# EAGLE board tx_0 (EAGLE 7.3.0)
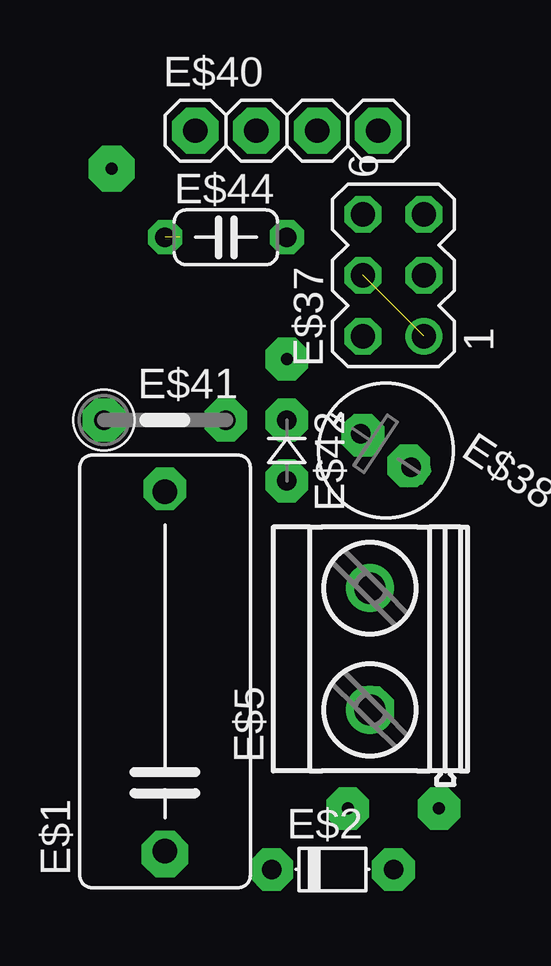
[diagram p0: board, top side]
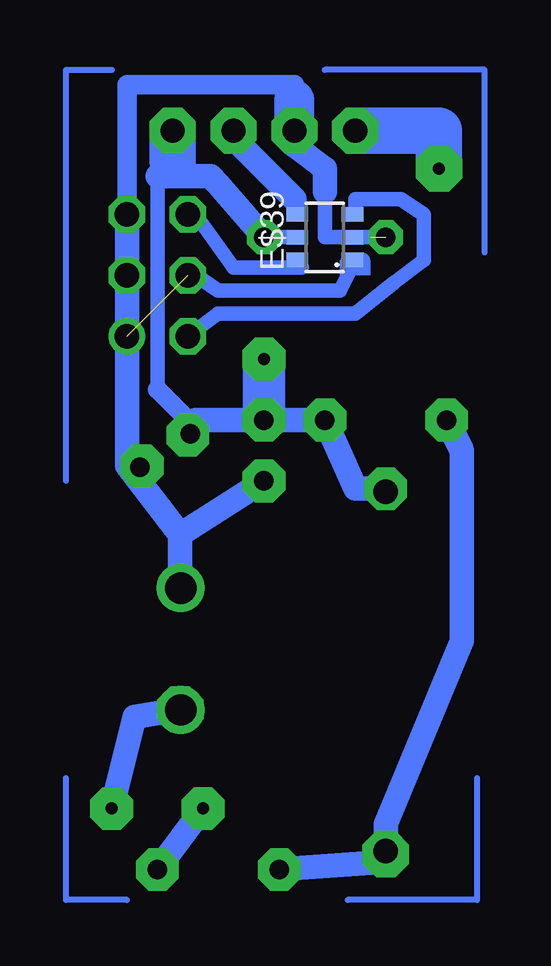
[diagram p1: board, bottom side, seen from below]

No outline drawn. Coordinates in mm, seen from the top.
Copper layers (1*16): Top 0.035mm / dielectric 1.5mm / Bottom 0.035mm
Design rules "default": minimum track width 10mil, minimum drill 24mil, track to track 8mil, track to pad 8mil, pad to pad 8mil, via to via 8mil, smd to smd 8mil, copper to edge 40mil, drill to drill 8mil, minimum pad ring 10mil, minimum via ring 8mil, stop-mask expansion 4mil, vias tented up to drill 0mil, thermal gap 10mil

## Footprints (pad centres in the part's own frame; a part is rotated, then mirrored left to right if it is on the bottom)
C150-072X183 = drill 1.016 octagon: 1 -7.493,0; 2 7.493,0
D-5 = drill 0.813 octagon: A 2.54,0; C -2.54,0
MKDSN1,5/2-5,08 = drill 1.3 pad 2: 1 -2.561,0.025; 2 2.519,0.025
MA03-2 = drill 1.016: 1 -2.54,-1.27 | drill 1.016 octagon: 2 -2.54,1.27; 3 0,-1.27; 4 0,1.27; 5 2.54,-1.27; 6 2.54,1.27
E2,5-6E = drill 0.813 pad 1.575: + -1.27,0 | drill 0.813 pad 1.575 octagon: - 1.27,0
SOT23-6 = smd 0.6 x 0.9: 1 -0.95,-1.15; 2 0,-1.15; 3 0.95,-1.15; 4 0.95,1.15; 5 0,1.15; 6 -0.95,1.15
1X04 = drill 1.016 octagon: 1 -3.81,0; 2 -1.27,0; 3 1.27,0; 4 3.81,0
0207/5V = drill 0.813 octagon: 1 -2.54,0; 2 2.54,0
D-2.5 = drill 0.813 octagon: A 1.27,0; C -1.27,0
C050-024X044 = drill 0.813 octagon: 1 -2.54,0; 2 2.54,0

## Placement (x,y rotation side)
E$1  [C150-072X183]  -13.02,27.94 90 top
E$2  [D-5]  -6.03,19.68 0 top
E$5  [MKDSN1,5/2-5,08]  -4.45,28.89 90 top
E$37  [MA03-2]  -3.49,44.45 90 top
E$38  [E2,5-6E]  -3.81,37.15 326.3 top
E$39  [SOT23-6]  -10.48,46.04 90 bottom
E$40  [1X04]  -7.94,50.48 0 top
E$41  [0207/5V]  -13.02,38.42 0 top
E$42  [D-2.5]  -7.94,37.15 270 top
E$44  [C050-024X044]  -10.48,46.04 0 top

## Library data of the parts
E$1 E$38 E$41 E$44 = rcl
E$2 E$42 = diode
E$5 = con-phoenix-508
E$37 = con-lstb
E$39 = microchip
E$40 = pinhead_hex

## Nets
S$128: E$37.6
S$129: E$37.4
S$130: E$37.2
S$139: E$38.+
S$158: E$42.A
S$162: E$37.5 E$38.-

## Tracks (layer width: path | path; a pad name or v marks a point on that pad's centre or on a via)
S$125
  Bottom 1.016: -15.56,38.42 -16.19,37.15 -16.19,29.21 -13.02,21.59 -13.02,20 -8.57,19.68
S$126  (via drill 0.5 pad 1.93)
  Bottom 1.93: v-15.24,48.9 -15.24,50.48 -11.75,50.48
S$127
  Bottom 0.61: -9.21,47.62 -9.21,46.99 | -6.67,50.16 -6.67,50.48
  Bottom 1.016: -9.21,47.62 -6.67,50.16
S$128
  Bottom 0.61: -9.53,44.77 -6.67,44.77 -5.08,46.99 E$37.6
S$129
  Bottom 0.61: -11.75,45.09 -11.11,43.81 -6.03,43.81 -5.08,44.45 E$37.4
S$130
  Bottom 0.61: -11.75,46.99 -11.75,47.62 -13.65,47.62 -14.61,46.99 -14.61,45.09 -13.34,44.13 -11.75,42.86 -6.03,42.86 E$37.2
S$131  (via drill 0.5 pad 1.93)
  other vias: -13.02,20.32
S$132  (via drill 0.5 pad 1.78, 0.5 pad 1.93)
  Bottom 1.016: v-4.45,26.35 -2.54,26.04 v-1.59,22.23
S$133  (via drill 0.5 pad 1.42)
  other vias: -4.76,41.91
S$135  (via drill 0.5 pad 1.78)
  other vias: -13.02,35.56
S$136  (via drill 0.5 pad 1.78)
  other vias: -10.48,38.42
S$137  (via drill 0.5 pad 1.78)
  other vias: -4.76,37.78
S$138  (via drill 0.5 pad 1.93)
  other vias: -6.67,50.48
S$139  (via drill 0.5 pad 1.93)
  Bottom 0.61: -3.49,39.69 -3.49,48.58 | -7.94,46.04 -9.21,46.04
  Bottom 0.813: -3.49,48.58 -4.13,48.58 -4.13,49.21 | -5.08,38.1 -3.49,39.69
  Bottom 1.016: -7.94,46.04 -6.03,48.26 -5.71,48.58 -3.49,48.58 | E$38.+ -5.08,38.1 -5.08,38.42 -10.48,38.42 -11.75,35.56 -13.02,35.56
  Bottom 1.778: -4.13,49.53 -4.13,49.21
  Bottom 1.93: -4.13,49.53 v-4.13,50.48 -4.13,49.21
S$140  (via drill 0.5 pad 1.93)
  other vias: -9.21,50.48
S$141  (via drill 0.5 pad 1.93)
  other vias: -11.75,50.48
S$142  (via drill 0.5 pad 1.42)
  other vias: -2.22,46.99
S$143  (via drill 0.5 pad 1.42)
  other vias: -4.76,46.99
S$144  (via drill 0.5 pad 1.42)  (1 unrouted)
  other vias: -4.76,44.45 -2.22,41.91
S$145  (via drill 0.5 pad 1.42)
  other vias: -2.22,44.45
S$146  (via drill 0.5 pad 1.42)
  other vias: -2.22,41.91
S$147  (via drill 0.5 pad 1.78)
  other vias: -2.86,36.51
S$148  (via drill 0.5 pad 1.78)
  other vias: -15.56,38.42
S$149  (via drill 0.5 pad 1.78)
  other vias: -4.45,31.43
S$151  (via drill 0.5 pad 1.78)
  Bottom 1.016: v-5.4,22.23 v-3.49,19.68
S$152  (via drill 0.5 pad 1.78)
  other vias: -8.57,19.68
S$153
  Bottom 0.254: -1.59,53.02 0.32,53.02 0.32,35.88
S$154
  Bottom 0.254: 0.32,23.5 0.32,18.41 -2.22,18.41
S$155
  Bottom 0.254: -10.48,53.02 -17.14,53.02 -17.14,45.4
S$156
  Bottom 0.254: -11.43,18.41 -16.83,18.41 -16.83,23.5
S$157  (via drill 0.5 pad 1.42)
  other vias: -7.94,46.04
S$158
  Bottom 1.016: E$42.A -4.45,33.66
S$159  (via drill 0.5 pad 1.78)
  other vias: -7.94,35.88
S$160  (via drill 0.5 pad 1.78)
  Bottom 1.778: v-7.94,40.96 v-7.94,38.42
S$161
  Bottom 0.61: -12.06,45.09 -11.43,45.09
S$162  (via drill 0.5 pad 1.42)  (1 unrouted)
  Bottom 0.61: -12.38,46.04 -10.48,46.04 -10.48,47.94
  Bottom 0.813: -9.21,51.75 -9.21,52.39 -2.22,52.39 E$37.5 | -9.21,50.48 -9.21,49.85
  Bottom 1.016: -9.21,49.85 -10.48,48.9 -10.48,47.94 | -2.22,36.51 E$37.5 | -2.22,36.51 E$38.- | -2.22,36.51 -4.45,33.66 -4.45,31.43
  Bottom 1.676: -9.21,50.48 -9.21,51.75
  other vias: -13.02,46.04
(copper drawn outside any net)
  shapes: Bottom area x1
